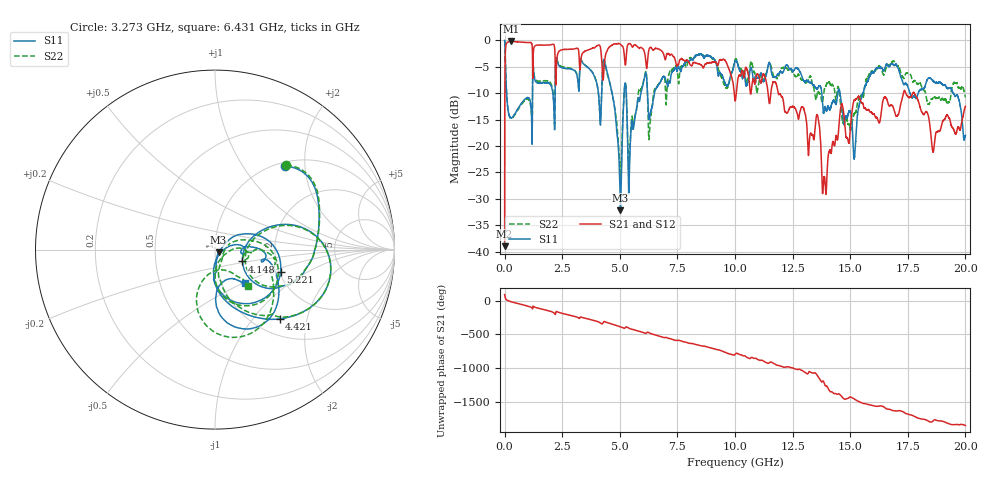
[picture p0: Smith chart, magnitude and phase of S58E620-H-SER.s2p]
!{S58E620}
!Johanson Technology Inc.
!www.johansontechnology.com
!Test Board Conditions:
!Substrate Type  RO4350B
!Substrate Thickness  60 mil
!Substrate Dk  3.66
!TL Type: GCPW
!TL Trace Width  115 mil
!TL Gap  52 mil
!Electrode orientation  Horizontal
!DUT TOPOLOGY	SERIES
!Mounting Pad LxW  55x428 mil
! Created Wed Apr 14 11:59:04 2021
# mhz S ma R 50
! 2 Port Network Data from SP1.SP block
! freq  magS11  angS11  magS21  angS21  magS12  angS12  magS22  angS22
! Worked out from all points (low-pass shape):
!   20001 points, 300 kHz to 20 GHz, reference 50 ohm
!   highest |S21| = -0.21 dB at 287.3 MHz (marker M1); lowest = -38.9 dB at 300 kHz (marker M2)
!   |S21| within 3 dB of the highest: 25.82 MHz to 1.211 GHz (1.186 GHz wide, 192 % of centre); 2.278 GHz to 3.236 GHz (958.3 MHz wide, 34.8 % of centre)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
!   lowest |S11| = -32.2 dB at 5.028 GHz (marker M3), VSWR 1.05, Z = 52 - j1.52 ohm
!   |S11| at or under -10 dB: 86.54 MHz to 1.211 GHz (1.124 GHz wide, 173 % of centre); 13.77 GHz to 14.46 GHz (695.4 MHz wide, 4.93 % of centre); 14.56 GHz to 15.55 GHz (988 MHz wide, 6.56 % of centre)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
!   |S22| runs from -26.0 to 0.0 dB; largest |S21 - S12| = 0.0084
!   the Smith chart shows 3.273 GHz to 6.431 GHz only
!   S11 on the Smith chart (normalised r, x): 3.273 GHz: 1.08, +1.57; 4.148 GHz: 1.35, -0.18; 4.421 GHz: 1.29, -1.38; 5.221 GHz: 2.04, -0.59; 6.431 GHz: 1.29, -0.52
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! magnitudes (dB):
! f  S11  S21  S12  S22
! 300 kHz  0.0  -38.9  -38.9  0.0
! 105.3 MHz  -11.2  -0.4  -0.4  -11.3
! 287.3 MHz  -14.7  -0.2  -0.2  -14.8
! 3.273 GHz  -4.4  -5.5  -5.5  -4.2
! 3.334 GHz  -3.8  -3.0  -3.0  -3.8
! 4.148 GHz  -15.6  -1.2  -1.2  -15.0
! 4.421 GHz  -5.5  -2.2  -2.2  -5.8
! 5.028 GHz  -32.2  -0.7  -0.7  -25.3
! 5.221 GHz  -8.3  -4.1  -4.1  -8.4
! 5.419 GHz  -24.4  -0.6  -0.6  -22.2
! 6.066 GHz  -7.2  -2.2  -2.1  -7.0
! 6.431 GHz  -12.0  -1.8  -1.8  -11.2
! 6.667 GHz  -8.5  -1.6  -1.6  -8.4
! 10 GHz  -3.9  -11.4  -11.3  -3.6
! 13.33 GHz  -8.0  -17.9  -17.9  -7.8
! 13.61 GHz  -8.9  -14.7  -14.6  -9.6
! 13.88 GHz  -13.0  -25.8  -25.9  -9.2
! 15.18 GHz  -22.3  -11.3  -11.3  -13.8
! 16.67 GHz  -4.9  -12.2  -12.5  -4.7
! 17.8 GHz  -10.6  -10.2  -10.1  -7.6
! 18.6 GHz  -7.6  -21.1  -21.1  -10.9
! 20 GHz  -17.9  -12.5  -12.5  -10.7
